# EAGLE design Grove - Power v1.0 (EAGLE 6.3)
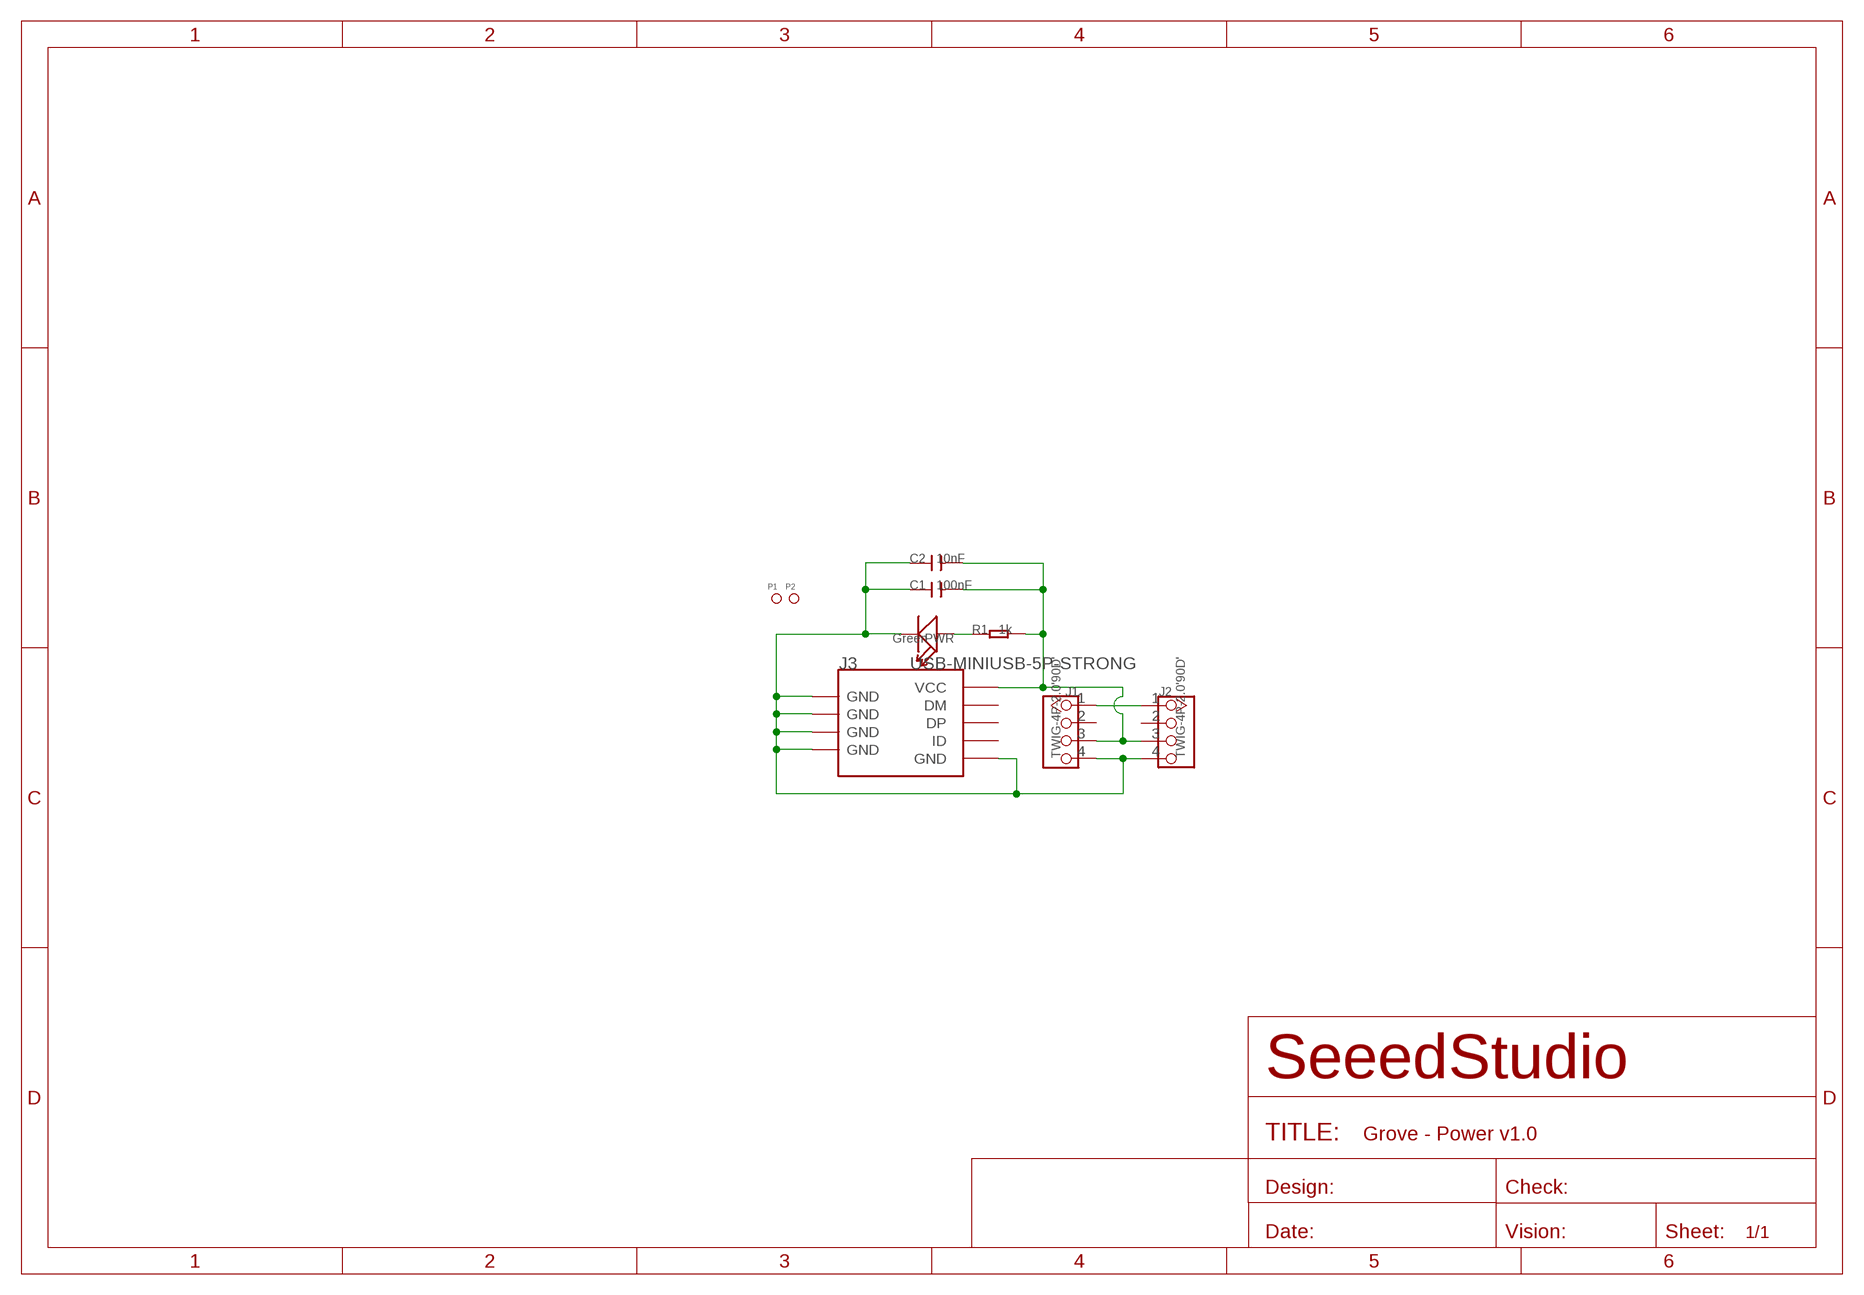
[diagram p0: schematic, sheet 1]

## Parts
C1  100nF  C-0603  [C0603]
C2  10nF  C-0603  [C0603]
J1  TWIG-4P-2.0'90D'  [4P-2.0-90D]
J2  TWIG-4P-2.0'90D'  [4P-2.0-90D]
J3  USB-MINIUSB-5P-STRONG  [MINI-SMD-5P]
P1  PAD-MARK  [ROUND-MARK-1.0]
P2  PAD-MARK  [ROUND-MARK-1.0]
PWR  Green  LED'0603'  [LED-0603]
R1  1k  R-0603  [R0603]

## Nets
GND: C1.1 C2.1 J1.4 J2.4 J3.5(GND) J3.GND@1(GND) J3.GND@2(GND) J3.GND@3(GND) J3.GND@4(GND) PWR.-
N$3: PWR.+ R1.1
SIG: J1.1 J2.1
VCC: C1.2 C2.2 J1.3 J2.3 J3.1(VCC) R1.2
Unconnected: J1.2 J2.2 J3.2(DM) J3.3(DP) J3.4(ID)

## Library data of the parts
C1 C2 = Discrete:C*: Ceramic Capacitors
J1 J2 = Connector:TWIG-4P-2.0
J3 = Connector:USB-MINIUSB-5P
P1 P2 = Discrete:PAD-MARK; PARTNO: DNP
PWR = Discrete:LED*
R1 = Discrete:R*

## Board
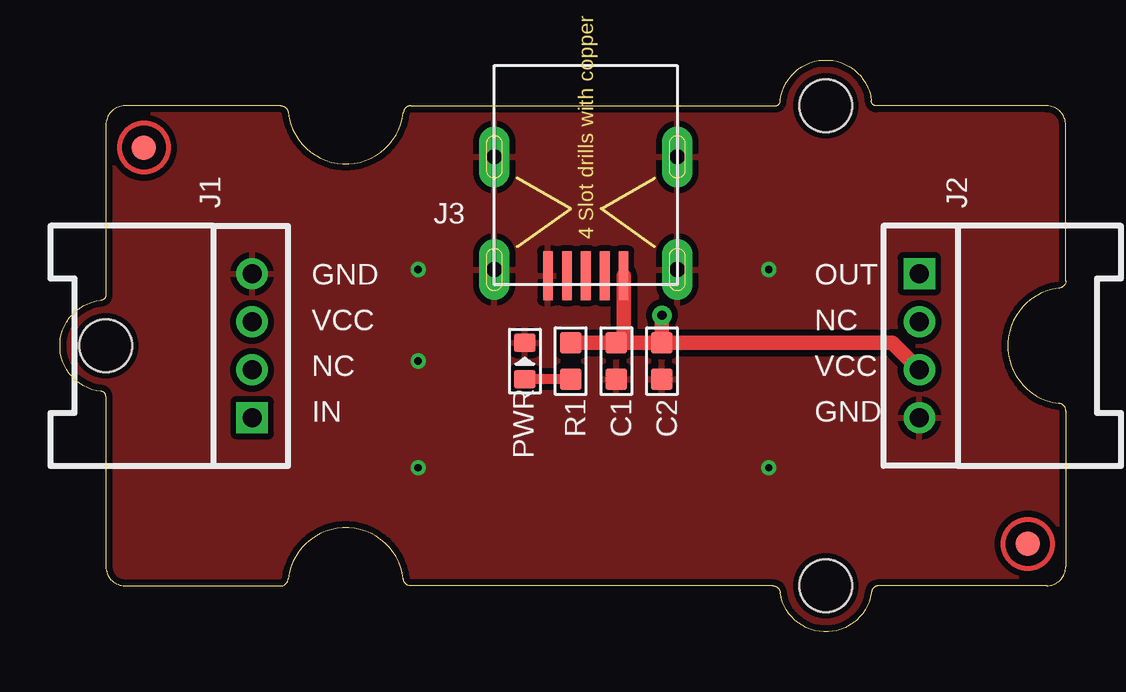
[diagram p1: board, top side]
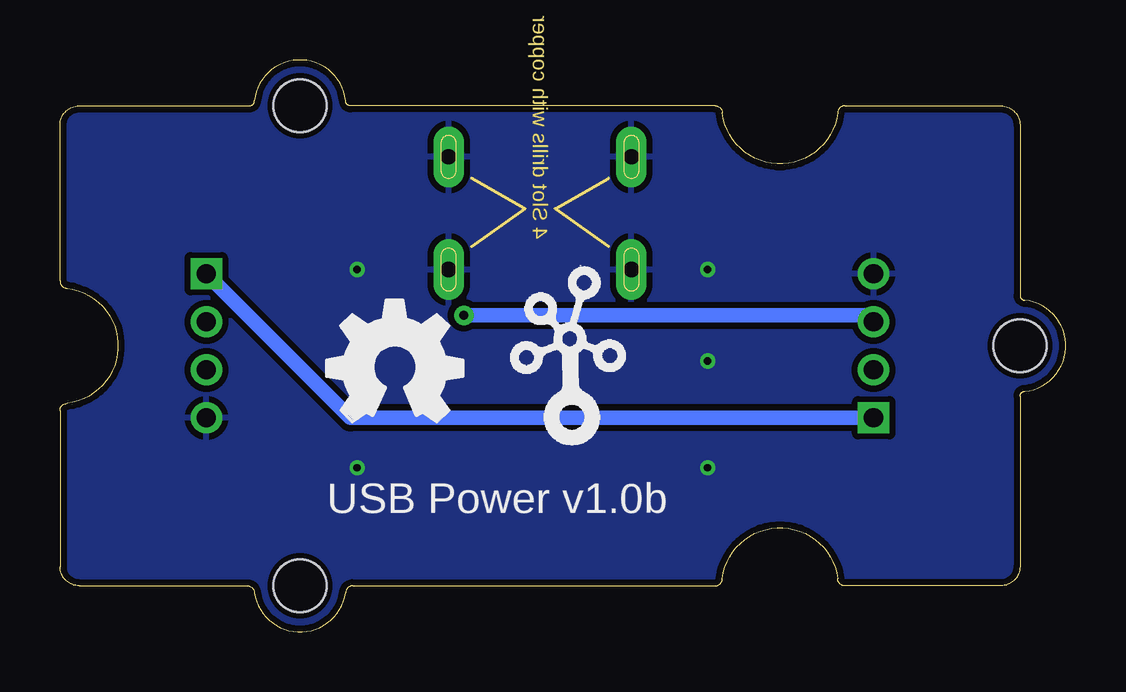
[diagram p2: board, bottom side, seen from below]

Size 41.91 x 23.83 mm. Coordinates in mm from the lower left corner, seen from the top.
Copper layers (1*16): Top 0.035mm / dielectric 1.5mm / Bottom 0.035mm
Design rules "SeeedStudio_rule_no_angle_090911 *": minimum track width 6mil, minimum drill 12mil, track to track 6mil, track to pad 6mil, pad to pad 6mil, via to via 6mil, smd to smd 0mil, copper to edge 10mil, drill to drill 10mil, minimum pad ring 10mil, minimum via ring 6mil, stop-mask expansion 2mil, vias tented up to drill 100mil, thermal gap 10mil

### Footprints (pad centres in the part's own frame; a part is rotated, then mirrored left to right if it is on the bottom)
C0603 = smd 0.889 x 0.889: 1 -0.762,0; 2 0.762,0
4P-2.0-90D = drill 0.8 pad 1.27 square: 1 -3,0 | drill 0.8 pad 1.27: 2 -1,0; 3 1,0; 4 3,0
MINI-SMD-5P = smd 2.032 x 0.406: 1 0.381,-1.575; 2 0.381,-0.787; 3 0.381,0; 4 0.381,0.787; 5 0.381,1.575 | drill 0.635 pad 1.27 long: GND@1 0.635,3.81; GND@2 5.334,3.81; GND@3 5.334,-3.81; GND@4 0.635,-3.81
ROUND-MARK-1.0 = smd 1.016 x 1.016: P$1 0,0
LED-0603 = smd 0.762 x 0.889: + -0.762,0; - 0.762,0
R0603 = smd 0.889 x 0.889: 1 -0.762,0; 2 0.762,0
2U-DIM-W/DRILL = hole 2.2: -10,-10; -10,10; 20,0

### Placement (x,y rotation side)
C1  23.18,11.29 90 top
C2  25.08,11.29 90 top
J1  8.01,11.92 90 top
J2  35.81,11.92 270 top
J3  21.91,14.46 90 top
P1  3.49,20.18 0 top
P2  40.32,3.67 0 top
PWR  19.37,11.29 90 top
R1  21.27,11.29 90 top
U$1  [2U-DIM-W/DRILL]  21.91,11.92 180 top
U$2  [OSHW_FILLX200_NOTEXT]  30.8,8.75 0 bottom
U$3  [TWIGLOGO]  20.64,8.75 0 bottom

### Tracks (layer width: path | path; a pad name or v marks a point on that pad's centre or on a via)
GND  (via drill 0.3 pad 0.64)
  other vias: 14.92,15.1 14.92,6.84 29.53,6.84 29.53,15.1 14.92,11.29
  pour Bottom (isolate 0.254): -0.32,-0.14 42.23,-0.14 42.23,23.99 -0.32,23.99
  pour Top (isolate 0.254): -0.32,-0.14 42.23,-0.14 42.23,23.99 -0.32,23.99
N$3
  Top 0.406: R1.1 PWR.+
SIG
  Bottom 0.61: J1.1 29.81,8.92 J2.1
VCC  (via drill 0.38 pad 0.81)
  Top 0.61: J3.1 23.48,12.35 C1.2 | R1.2 C1.2 | C2.2 C1.2 | C2.2 34.68,12.05 J2.3 | C2.2 v25.08,13.19
  Bottom 0.61: v25.08,13.19 8.28,13.19 J1.3

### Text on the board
tPlace: GND | OUT | VCC | NC | NC | VCC | IN | GND
bPlace: USB Power v1.0b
